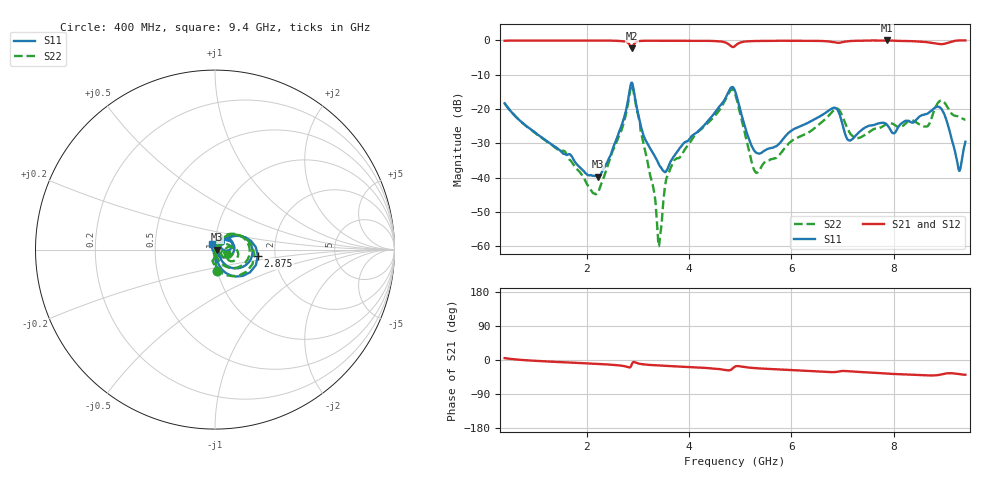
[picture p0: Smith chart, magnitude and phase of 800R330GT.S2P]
!  American Technical Ceramics  Date:  6/19/09
!  One Norden Lane
!  Huntington Station,  NY.  11746-2102
!  Tel:  (631) 622-4700  Fax:  (631) 622-4748
!  Part Number  800R330GT
!  Description: Ultra-low ESR, NPO  Mounting Orientation: Horizontal
!  Application: High RF power Filters, Combiners, Matching networks,
!  Antenna, DC block, Bypass and Couplers
# GHZ S DB R 50
! Freq  |S11|  S11 Ph  |S21|  S21 Ph  |S12|  S12 Ph  |S22|  S22 Ph
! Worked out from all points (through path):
!   801 points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, 400 MHz to 9.4 GHz, reference 50 ohm
!   highest |S21| = 0.00 dB at 7.87 GHz (marker M1); lowest = -2.3 dB at 2.886 GHz (marker M2)
!   group delay of S21, straight-line fit = 12.7 ps
!   lowest |S11| = -39.8 dB at 2.223 GHz (marker M3), VSWR 1.02, Z = 51 - j0.122 ohm
!   |S11| at or under -10 dB: start of sweep to end of sweep
!   |S22| runs from -60.0 to -13.0 dB; largest |S21 - S12| = 0.0023
!   S11 on the Smith chart (normalised r, x): 400 MHz: 1.00, -0.24; 2.875 GHz: 1.62, -0.12; 9.4 GHz: 0.97, +0.06
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0.4  -18.32 -84.0  -0.08 5.0  -0.09 5.1  -18.32 -84.5
1.908  -37.55 -62.0  -0.03 -8.2  -0.04 -8.2  -39.20 -119.0
2.223  -39.75 -6.7  -0.04 -10.3  -0.05 -10.3  -44.33 146.9
2.628  -27.03 48.0  -0.13 -14.2  -0.14 -14.1  -28.03 73.1
2.875  -12.34 -8.2  -2.29 -14.6  -2.30 -14.6  -13.09 -7.1
2.886  -12.27 -20.9  -2.30 -10.6  -2.31 -10.6  -12.99 -21.2
3.303  -32.92 -54.9  -0.09 -13.6  -0.09 -13.6  -42.83 -85.4
3.404  -35.78 -41.9  -0.07 -14.4  -0.08 -14.4  -59.96 -30.5
3.449  -36.91 -30.0  -0.07 -14.7  -0.07 -14.7  -55.71 54.0
3.561  -38.02 8.3  -0.06 -15.7  -0.06 -15.6  -40.18 86.8
3.696  -33.98 32.5  -0.08 -16.6  -0.09 -16.6  -35.36 78.2
4.9  -14.70 -31.1  -1.62 -17.4  -1.63 -17.3  -15.53 -34.6
5.316  -32.71 -15.3  -0.16 -21.7  -0.16 -21.6  -38.62 -20.0
6.408  -23.35 54.7  -0.12 -29.1  -0.12 -29.0  -26.12 37.1
6.88  -19.84 15.9  -0.66 -31.4  -0.65 -31.3  -19.85 -7.2
7.128  -29.16 22.3  -0.20 -29.8  -0.20 -29.7  -26.58 -39.5
7.87  -24.60 35.2  0.00 -35.8  -0.01 -35.7  -24.30 -13.2
7.904  -25.26 33.8  -0.01 -36.1  -0.01 -36.1  -24.13 -15.7
8.635  -21.45 37.1  -0.47 -40.8  -0.46 -40.8  -25.12 -7.2
8.871  -19.31 3.9  -1.00 -39.7  -0.99 -39.6  -18.04 -3.8
9.265  -37.41 -124.2  -0.01 -37.2  -0.01 -37.1  -22.30 -28.1
9.4  -29.55 115.9  -0.01 -38.9  -0.01 -38.8  -23.02 -18.0
